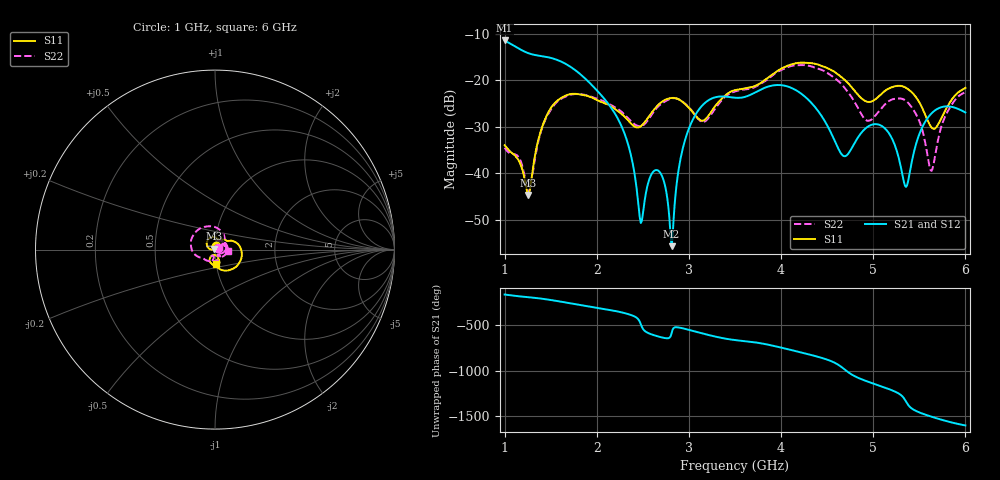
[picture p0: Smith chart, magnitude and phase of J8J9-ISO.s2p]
!Agilent Technologies,E8364B,MY43040528,A.07.50.67
!Agilent E8364B: A.07.50.67
!Date: Sunday, March 01, 2026 21:37:41
!Correction: S11(Full 2 Port(1,2))
!S21(Full 2 Port(1,2))
!S12(Full 2 Port(1,2))
!S22(Full 2 Port(1,2))
!S2P File: Measurements: S11, S21, S12, S22:
# Hz S  dB  R 50
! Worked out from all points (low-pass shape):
!   451 points, 1 GHz to 6 GHz, reference 50 ohm
!   highest |S21| = -11.44 dB at 1 GHz (marker M1); lowest = -55.7 dB at 2.811 GHz (marker M2)
!   |S21| within 3 dB of the highest: start of sweep to 1.3 GHz
!   lowest |S11| = -44.7 dB at 1.256 GHz (marker M3), VSWR 1.01, Z = 49.7 + j0.491 ohm
!   |S11| at or under -10 dB: start of sweep to end of sweep
!   |S22| runs from -44.0 to -16.7 dB; largest |S21 - S12| = 0.00087
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1e9  -34.00 67.2  -11.44 -169.5  -11.46 -169.5  -34.55 19.3
1.255556e9  -44.70 122.0  -14.17 161.5  -14.20 161.5  -43.99 59.0
1.488889e9  -26.43 154.9  -15.13 132.9  -15.15 132.9  -26.75 80.4
1.844444e9  -23.15 92.3  -19.10 72.1  -19.12 72.2  -23.07 -0.8
2.277778e9  -27.42 56.1  -30.32 -6.0  -30.33 -6.0  -26.95 -61.9
2.477778e9  -29.91 75.4  -50.75 -132.8  -50.76 -132.7  -29.89 -56.4
2.666667e9  -25.32 78.6  -39.47 93.0  -39.50 93.0  -25.65 -56.9
2.744444e9  -24.19 68.6  -43.03 74.8  -43.06 74.7  -24.52 -70.5
2.811111e9  -23.83 58.2  -55.74 125.1  -55.76 125.5  -23.92 -83.8
2.911111e9  -24.38 44.1  -36.68 -172.9  -36.71 -172.9  -24.36 -102.3
3.033333e9  -26.69 34.6  -28.85 156.2  -28.88 156.2  -26.60 -118.6
3.166667e9  -28.60 52.7  -25.01 120.8  -25.05 120.9  -28.94 -107.6
3.5e9  -22.13 46.1  -23.77 53.7  -23.80 53.7  -22.42 -124.8
4e9  -17.53 12.5  -21.06 -28.3  -21.09 -28.3  -17.81 -178.9
4.344444e9  -16.37 -38.1  -25.23 -113.6  -25.25 -113.6  -17.13 114.0
4.677778e9  -19.71 -80.8  -36.31 102.3  -36.35 102.3  -21.34 51.3
4.933333e9  -24.63 -78.6  -30.11 -36.9  -30.14 -36.9  -28.70 43.0
5.166667e9  -21.80 -74.8  -31.30 -120.1  -31.34 -120.1  -24.53 41.2
5.355556e9  -21.63 -101.9  -42.99 103.5  -43.03 103.6  -24.44 -1.3
5.633333e9  -30.19 -105.9  -27.12 -63.0  -27.16 -62.9  -39.53 7.1
5.777778e9  -26.65 -67.6  -25.65 -106.0  -25.69 -106.0  -27.89 38.7
6e9  -21.65 -85.6  -26.94 -157.9  -26.97 -157.9  -22.55 -4.0
